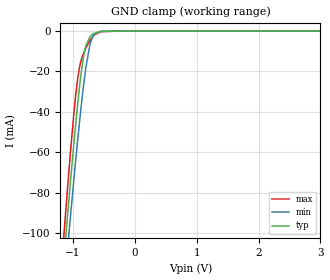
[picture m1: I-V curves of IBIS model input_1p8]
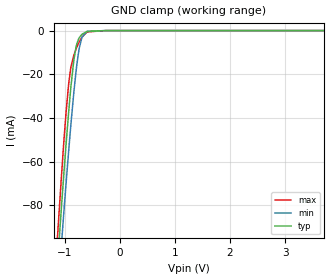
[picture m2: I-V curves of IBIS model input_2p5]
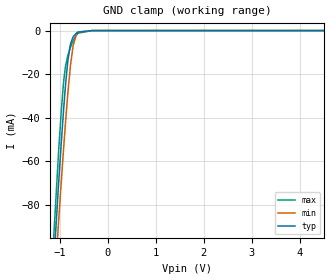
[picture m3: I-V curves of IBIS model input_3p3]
|Texas Instruments Incorporated
| Low Voltage 2-Channel I2C Bus Switch With Interrupt Logic And Reset
| Marketing part#   Digital Voltage Range   Package-type   #pins
| TCA9543APWR   1.65V-5.5V   TSSOP   14
[IBIS Ver]   4.1
[File name]   tca9543a.ibs
[File Rev]   1.0
[Date]   11/25/2013
[Source]
| Texas Instruments Incorporated.
| Analog-eLab Design Center, HPA
| 12500 TI Blvd
| Dallas, TX -75243
[Notes]   Revision History:
| Rev 1.0: 11/25/2013
| - Initial version of the model
| - Model generated from simulations in TISPICE
| - Model matched to SPICE simulation
| - C_comp although listed in numerical order of value are
|   obtained from varying PVT conditions. For PVT conditions for
|   each specific value refer the buffer description under
|   respective [Model]. IBIS model user is responsible for using
|   appropriate C_comp to simulate for Signal Integrity.
|*  EXCEPTION:   *
|*  - For model input_5p0, scl_5p0 and sda_5p0,there will be a surge   *
|*   current in the GROUND clamp I-V Table because of the four switches *
|*   (SWITCH) connected to the pad.   *
[Disclaimer]
| This model is designed as an aid for customers of Texas Instruments.
| TI and its licensors and suppliers make no warranties, either expressed
| or implied, with respect to this  model, including the warranties of
| merchantability or fitness for a particular purpose. The model is
| provided solely on an "as is" basis. The entire risk as to its quality
| and performance is with the customer.
[Copyright]
(C) Copyright 2013 Texas Instruments Incorporated.All rights reserved.
|   TCA9543A
[Component]   TCA9543A
[Manufacturer]   TI
[Package]   |14 TSSOP  -  PW package
|   typ   min   max
R_pkg   0.18301   0.17482   0.20104
L_pkg   3.37880nH   3.14028nH   3.98755nH
C_pkg   0.48842pF   0.47332pF   0.53955pF
[Pin]  signal_name   model_name   R_pin   L_pin   C_pin
1   A0   NC   0.18817   3.98843nH  0.54185pF
2   A1   NC   0.20582   3.55611nH  0.49573pF
3   _RESET   INPUT   0.17978   3.24464nH  0.47374pF
4   _INT0   INPUT   0.17482   3.14028nH  0.47332pF
5   SD0   NC   0.18010   3.25061nH  0.47698pF
6   SC0   NC   0.19395   3.45427nH  0.48953pF
7   GND   GND   0.18497   3.96444nH  0.53743pF
8   _INT1   INPUT   0.18740   3.98755nH  0.53955pF
9   SD1   NC   0.19502   3.46498nH  0.49070pF
10   SC1   NC   0.18032   3.25120nH  0.47494pF
11   _INT   INTZ   0.17546   3.14519nH  0.47380pF
12   SCL   SCL   0.17957   3.24286nH  0.47592pF
13   SDA   SDA   0.20104   3.51227nH  0.49419pF
14   VCC   POWER   0.18754   3.98375nH  0.54135pF
|   Model Selectors
[Model Selector] INPUT
input_1p8   1.8V  digital input
input_2p5   2.5V  digital input
input_3p3   3.3V  digital input
input_5p0   5.0V  digital input
[Model Selector] SCL
scl_1p8   1.8V  digital input
scl_2p5   2.5V  digital input
scl_3p3   3.3V  digital input
scl_5p0   5.0V  digital input
[Model Selector] INTZ
intz_1p8   1.8V  digital Open_drain
intz_2p5   2.5V  digital Open_drain
intz_3p3   3.3V  digital Open_drain
intz_5p0   5.0V  digital Open_drain
[Model Selector] SDA
sda_1p8   1.8V  digital I/O_open_drain
sda_2p5   2.5V  digital I/O_open_drain
sda_3p3   3.3V  digital I/O_open_drain
sda_5p0   5.0V  digital I/O_open_drain
| Models and submodels in the file (16): input_1p8 (Input), input_2p5 (Input), input_3p3 (Input), input_5p0 (Input), scl_1p8 (Input), scl_2p5 (Input), scl_3p3 (Input), scl_5p0 (Input), intz_1p8 (Open_drain), intz_2p5 (Open_drain), intz_3p3 (Open_drain), intz_5p0 (Open_drain), sda_1p8 (I/O_open_drain), sda_2p5 (I/O_open_drain), sda_3p3 (I/O_open_drain), sda_5p0 (I/O_open_drain)
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|   input_1p8 Model
[Model]   input_1p8
Model_type   Input
Vinl = 0.54
Vinh = 1.26
|   typ   min   max
|   (nom PVT)   (fast PVT)   (slow PVT)
C_comp   1.378e-12   1.328e-12   1.458e-12
[Model spec]
|subparameter
Vinl   0.54   0.504   0.594
Vinh   1.26   1.176   1.386
| Where nom  PVT is Nominal Process, 1.8V, 27C
|   Fast PVT is Strong Process,  1.98V, -40C
|   Slow PVT is Weak Process,   1.68V, 85C
[Voltage Range]   1.8   1.68   1.98
|Junction Temperature
[Temperature Range]   27   85   -40
[Power Clamp Reference]   1.8   1.68   1.98
[GND Clamp Reference]   0   0   0
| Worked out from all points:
|   GND clamp passes 1 mA (typ) near -0.64 V on its own axis
[GND Clamp]
|   Voltage   I(typ)   I(min)   I(max)
-1.8V     -375.9mA   -377.1mA   -385mA
-1.168V   -121.8mA   -137.1mA   -110.5mA
-1.117V   -102.7mA   -118.9mA   -89.99mA
-1.052V   -79.45mA   -96.6mA    -65.26mA
-953.3mV  -45.93mA   -63.89mA   -31.72mA
-887.2mV  -26.39mA   -43.66mA   -17.18mA
-843.7mV  -15.94mA   -31.43mA   -12.29mA
-788.4mV  -7.196mA   -17.96mA   -8.275mA
-728.2mV  -3.028mA   -7.407mA   -4.891mA
-669.4mV  -1.377mA   -2.257mA   -2.468mA
-180mV    -11.16nA   -21.74nA   0A
3.6V      0A         0A         0A
[POWER Clamp]
|   Voltage   I(typ)   I(min)   I(max)
-1.8V     0A         0A         0A
-1.615V   0A         0A         0A
3.6V      0A         0A         0A
|   input_2p5 Model
[Model]   input_2p5
Model_type   Input
Vinl = 0.75
Vinh = 1.75
|   typ   min   max
|   (nom PVT)   (fast PVT)   (slow PVT)
C_comp   1.365e-12   1.316e-12   1.458e-12
[Model spec]
|subparameter
Vinl   0.75   0.675   0.825
Vinh   1.75   1.575   1.925
| Where nom  PVT is Nominal Process, 2.5V, 27C
|   Fast PVT is Strong Process,  2.75V, -40C
|   Slow PVT is Weak Process,   2.25V, 85C
[Voltage Range]   2.5   2.25   2.75
|Junction Temperature
[Temperature Range]   27   85   -40
[Power Clamp Reference]   2.5   2.25   2.75
[GND Clamp Reference]   0   0   0
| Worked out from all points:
|   GND clamp passes 1 mA (typ) near -0.64 V on its own axis
[GND Clamp]
|   Voltage   I(typ)   I(min)   I(max)
-2.5V     -675.8mA   -660.2mA   -706.6mA
-1.14V    -111.3mA   -127mA     -99.14mA
-1.059V   -81.79mA   -98.85mA   -67.72mA
-1.025V   -69.86mA   -87.34mA   -55.26mA
-925mV    -37.17mA   -55.03mA   -24.34mA
-883mV    -25.27mA   -42.43mA   -16.57mA
-830.7mV  -13.4mA    -28.04mA   -11.23mA
-792.5mV  -7.656mA   -18.85mA   -8.537mA
-731.5mV  -3.168mA   -7.851mA   -5.056mA
-685mV    -1.706mA   -3.181mA   -3.022mA
-600mV    -476.3uA   -460.6uA   -817.6uA
5V        0A         0A         0A
[POWER Clamp]
|   Voltage   I(typ)   I(min)   I(max)
-2.5V     0A         0A         0A
-2.392V   0A         0A         0A
5V        0A         0A         0A
|   input_3p3 Model
[Model]   input_3p3
Model_type   Input
Vinl = 0.99
Vinh = 2.31
|   typ   min   max
|   (nom PVT)   (fast PVT)   (slow PVT)
C_comp   1.359e-12   1.298e-12   1.458e-12
[Model spec]
|subparameter
Vinl   0.99   0.9   1.08
Vinh   2.31   2.1   2.52
| Where nom  PVT is Nominal Process, 3.3V, 27C
|   Fast PVT is Strong Process,  3.6V, -40C
|   Slow PVT is Weak Process,   3V, 85C
[Voltage Range]   3.3   3   3.6
|Junction Temperature
[Temperature Range]   27   85   -40
[Power Clamp Reference]   3.3   3   3.6
[GND Clamp Reference]   0   0   0
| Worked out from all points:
|   GND clamp passes 1 mA (typ) near -0.65 V on its own axis
[GND Clamp]
|   Voltage   I(typ)   I(min)   I(max)
-3.3V     -1.027A    -992.8mA   -1.081A
-1.165V   -120.7mA   -136mA     -109.2mA
-1.036V   -73.54mA   -90.91mA   -59.08mA
-974.4mV  -52.76mA   -70.66mA   -38.09mA
-927.3mV  -37.86mA   -55.74mA   -24.88mA
-881.1mV  -24.77mA   -41.88mA   -16.31mA
-831.6mV  -13.56mA   -28.26mA   -11.3mA
-782.1mV  -6.544mA   -16.62mA   -7.881mA
-723mV    -2.826mA   -6.756mA   -4.642mA
-621mV    -671.7uA   -744.6uA   -1.186mA
-330mV    -1.205uA   -1.156uA   -944.2nA
6.6V      0A         0A         0A
[POWER Clamp]
|   Voltage   I(typ)   I(min)   I(max)
-3.3V     0A         0A         0A
-3.243V   0A         0A         0A
6.6V      0A         0A         0A
